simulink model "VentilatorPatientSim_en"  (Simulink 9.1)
settings: Solver=ode3  StartTime=0.0  StopTime=45  FixedStep=0.0001  RelTol=1e-3  EnableMultiTasking=on
undefined symbols (not defined in the file or in its folder): sgn

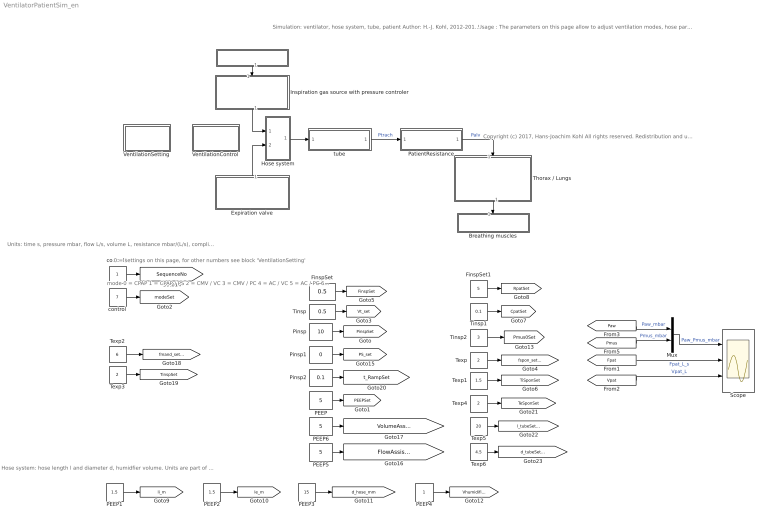
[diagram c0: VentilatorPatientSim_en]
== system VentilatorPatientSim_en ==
  note: Usage : The parameters on this page allow to adjust ventilation modes, hose parameters and patient properties. SequenceNo can select preprogrammed sequences. Suggestions : - place monitors at signals of interest - program a leak simulation and a leak compensation by the ventilator
  note: Copyright (c) 2017, Hans-Joachim Kohl All rights reserved. Redistribution and use in source and binary forms, with or without modification, are permitted provided that the following conditions are met: 1. Redistributions of source code must retain the above copyright notice, this list of conditions and the following disclaimer. 2. Redistributions in binary form must reproduce the above copyright notice, this list of conditions and the following disclaimer in the documentation and/or other materials provided with the distribution. THIS SOFTWARE IS PROVIDED BY THE COPYRIGHT HOLDERS AND CONTRIBUTORS "AS IS" AND ANY EXPRESS OR IMPLIED WARRANTIES, INCLUDING, BUT NOT LIMITED TO, THE IMPLIED WARRANTIES OF MERCHANTABILITY AND FITNESS FOR A PARTICULAR PURPOSE ARE DISCLAIMED. IN NO EVENT SHALL THE COPYRIGHT OWNER OR CONTRIBUTORS BE LIABLE FOR ANY DIRECT, INDIRECT, INCIDENTAL, SPECIAL, EXEMPLARY, OR CONSEQUENTIAL DAMAGES (INCLUDING, BUT NOT LIMITED TO, PROCUREMENT OF SUBSTITUTE GOODS OR SERVICES; LOSS OF USE, DATA, OR PROFITS; OR BUSINESS INTERRUPTION) HOWEVER CAUSED AND ON ANY THEORY OF LIABILITY, WHETHER IN CONTRACT, STRICT LIABILITY, OR TORT (INCLUDING NEGLIGENCE OR OTHERWISE) ARISING IN ANY WAY OUT OF THE USE OF THIS SOFTWARE, EVEN IF ADVISED OF THE POSSIBILITY OF SUCH DAMAGE. This is a simplified BSD license.
  note: Units: time s, pressure mbar, flow L/s, volume L, resistance mbar/(L/s), compliance L/mbar
  note: Hose system: hose length l and diameter d, humidfier volume. Units are part of the name.
  note: 0 = settings on this page, for other numbers see block 'VentilationSetting'
  note: mode 0 = CPAP 1 = CPAP / PS 2 = CMV / VC 3 = CMV / PC 4 = AC / VC 5 = AC / PC 6 = SIMV / VC 7 = SIMV / PC 8 = CPAP / ATC 9 = CPAP / PPS
  note: Simulation: ventilator, hose system, tube, patient Author: H.-J. Kohl, 2012-2019. Translation of a contribution 'Künstliche Beatmung' in 'Medizintechnische Systeme, ('Artificial Ventilation' in 'Medical Technology Systems') Springer Vieweg, ISBN 978-3-642-41238-7. The figures about ventilation modes have been created with this simulation. Technical details of the simulation are explained in a translated version of the contribution. Tested with Matlab 2017a
  " " : Subsystem
  Breathing muscles : Subsystem
  Expiration valve : Subsystem
  FinspSet : Constant  Value=0.5
  FinspSet1 : Constant  Value=5
  Hose system : Subsystem
  Inspiration gas source with pressure controler : Subsystem
  Mux : Mux  Inputs=2
  PEEP : Constant  Value=5
  PEEP1 : Constant  Value=1.5
  PEEP2 : Constant  Value=1.5
  PEEP3 : Constant  Value=15
  PEEP4 : Constant
  PEEP5 : Constant  Value=5
  PEEP6 : Constant  Value=5
  PatientResistance : Subsystem
  Pinsp : Constant  Value=10
  Pinsp1 : Constant  Value=0
  Pinsp2 : Constant  Value=0.1
  Scope : Scope  NumInputPorts=3
  Texp : Constant  Value=2
  Texp1 : Constant  Value=1.5
  Texp2 : Constant  Value=6
  Texp3 : Constant  Value=2
  Texp4 : Constant  Value=2
  Texp5 : Constant  Value=20
  Texp6 : Constant  Value=4.5
  Thorax / Lungs : Subsystem
  Tinsp : Constant  Value=0.5
  Tinsp1 : Constant  Value=0.1
  Tinsp2 : Constant  Value=3
  VentilationControl : Subsystem
  VentilationSetting : Subsystem
  control : Constant  Value=7  OutDataTypeStr=uint8
  control1 : Constant  OutDataTypeStr=uint32  SampleTime=0.0001
  tube : Subsystem
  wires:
  Thorax / Lungs/1(Pmus) -> Breathing muscles/1(" ")
  PatientResistance/1(" ") -> Thorax / Lungs/1(Palv)  "Palv"
  Pinsp/1 -> [PinspSet]
  PEEP/1 -> [PEEPSet]
  control/1 -> [modeSet]
  Tinsp/1 -> [Vt_set]
  Texp/1 -> [fspon_set_bpm]
  FinspSet/1 -> [FinspSet]
  Texp1/1 -> [TiSponSet]
  Tinsp1/1 -> [CpatSet]
  FinspSet1/1 -> [RpatSet]
  Inspiration gas source with pressure controler/1(Finsp) -> Hose system/1("   ")
  Expiration valve/1(" sValve") -> Hose system/2(" ")
  Hose system/1(Paw) -> tube/1(Paw)
  PEEP1/1 -> [li_m]
  PEEP2/1 -> [le_m]
  PEEP3/1 -> [d_hose_mm]
  PEEP4/1 -> [Vhumidifier_L]
  Tinsp2/1 -> [Pmus0Set]
  control1/1 -> [SequenceNo]
  Pinsp1/1 -> [PS_set]
  PEEP5/1 -> [FlowAssistSet_mbar__L_s]
  PEEP6/1 -> [VolumeAssistSet_mbar_L]
  Texp2/1 -> [fmand_set_bpm]
  Texp3/1 -> [TinspSet]
  Pinsp2/1 -> [t_RampSet]
  Texp4/1 -> [TeSponSet]
  tube/1(" ") -> PatientResistance/1(Ptrach)  "Ptrach"
  Texp5/1 -> [l_tubeSet_cm]
  Texp6/1 -> [d_tubeSet_mm]
  " "/1(" ") -> Inspiration gas source with pressure controler/1(" ")
  [Fpat] -> Scope/2  "Fpat_L_s"
  [Vpat] -> Scope/3  "Vpat_L"
  Mux/1 -> Scope/1  "Paw_Pmus_mbar"
  [Paw] -> Mux/1  "Paw_mbar"
  [Pmus] -> Mux/2  "Pmus_mbar"

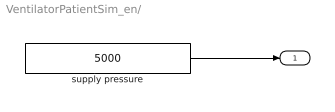
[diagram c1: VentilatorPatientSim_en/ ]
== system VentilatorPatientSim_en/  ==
  supply pressure : Constant  Value=5000
  " " : Outport
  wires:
  supply pressure/1 -> " "/1

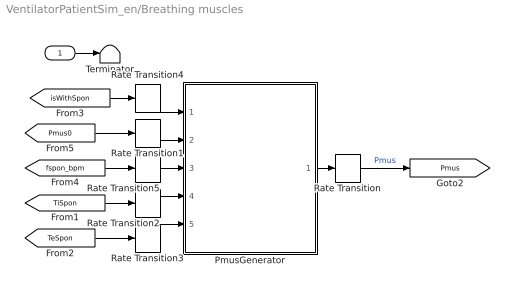
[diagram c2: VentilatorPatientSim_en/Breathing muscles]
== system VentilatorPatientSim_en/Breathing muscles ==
  " " : Inport
  PmusGenerator : Stateflow chart  TreatAsAtomicUnit=on
  Rate Transition{,1..5} (6 alike) : RateTransition  Integrity=off  Deterministic=off
  Terminator : Terminator
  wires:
  " "/1 -> Terminator/1
  PmusGenerator/1(Pmus) -> Rate Transition/1
  [TiSpon] -> Rate Transition2/1
  [TeSpon] -> Rate Transition3/1
  [Pmus0] -> Rate Transition1/1
  Rate Transition/1 -> [Pmus]  "Pmus"
  Rate Transition1/1 -> PmusGenerator/2(Pmus0)
  Rate Transition2/1 -> PmusGenerator/4(TiSpon)
  Rate Transition3/1 -> PmusGenerator/5(TeSpon)
  [isWithSpon] -> Rate Transition4/1
  Rate Transition4/1 -> PmusGenerator/1(isWithSpon)
  [fspon_bpm] -> Rate Transition5/1
  Rate Transition5/1 -> PmusGenerator/3(fspon_bpm)

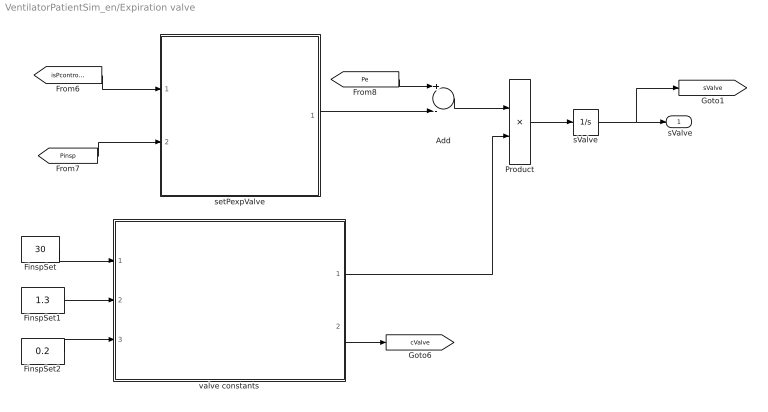
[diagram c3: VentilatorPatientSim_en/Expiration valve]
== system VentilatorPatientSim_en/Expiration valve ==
  Add : Sum  Inputs=+-
  FinspSet : Constant  Value=30
  FinspSet1 : Constant  Value=1.3
  FinspSet2 : Constant  Value=0.2
  Product : Product  Inputs=**
  sValve : Integrator  LimitOutput=on  UpperSaturationLimit=3  LowerSaturationLimit=0  ContinuousStateAttributes='sVentil'
  setPexpValve : Stateflow chart  TreatAsAtomicUnit=on
  valve constants : Stateflow chart  TreatAsAtomicUnit=on
  " sValve" : Outport
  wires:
  [isPcontrolled] -> setPexpValve/1(isPcontrolled)
  [Pinsp] -> setPexpValve/2(Pinsp)
  sValve/1 -> " sValve"/1, [sValve]
  [Pe] -> Add/1
  setPexpValve/1(PexpValve) -> Add/2
  Product/1 -> sValve/1
  Add/1 -> Product/1
  valve constants/1(cValve_sdot_mm_s__mbar) -> Product/2
  valve constants/2(cValve_flow_L_s__mm___mbar05) -> [cValve]
  FinspSet/1 -> valve constants/1(D_Valve_mm)
  FinspSet1/1 -> valve constants/2(rhoAir_kg_m3)
  FinspSet2/1 -> valve constants/3(tau3mm_s)

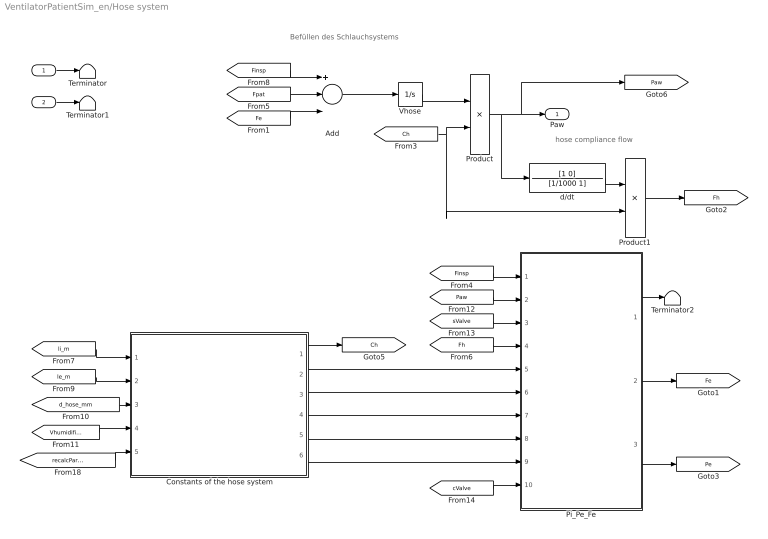
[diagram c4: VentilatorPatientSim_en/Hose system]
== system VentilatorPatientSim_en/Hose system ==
  note: Befüllen des Schlauchsystems
  note: hose compliance flow
  "   " : Inport
  " " : Inport  Port=2
  Add : Sum  Inputs=+--
  Constants of the hose system : Stateflow chart  TreatAsAtomicUnit=on
  Pi_Pe_Fe : Stateflow chart  TreatAsAtomicUnit=on
  Product : Product  Inputs=*/
  Product1 : Product
  Terminator : Terminator
  Terminator1 : Terminator
  Terminator2 : Terminator
  Vhose : Integrator
  d/dt : TransferFcn  Numerator=[1 0]  Denominator=[1/1000 1]
  Paw : Outport
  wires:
  "   "/1 -> Terminator/1
  " "/1 -> Terminator1/1
  [Finsp] -> Add/1
  Vhose/1 -> Product/1
  [Ch] -> Product/2, Product1/2
  Product/1 -> Paw/1, [Paw], d/dt/1
  Product1/1 -> [Fh]
  [Finsp] -> Pi_Pe_Fe/1(Finsp)
  [Fh] -> Pi_Pe_Fe/4(Fh)
  Pi_Pe_Fe/1(Pi) -> Terminator2/1
  Pi_Pe_Fe/2(Fe) -> [Fe]
  Pi_Pe_Fe/3(Pe) -> [Pe]
  Constants of the hose system/2(i_ie_Ch) -> Pi_Pe_Fe/5(i_ie_Ch)
  [li_m] -> Constants of the hose system/1(Li_m)
  [le_m] -> Constants of the hose system/2(Le_m)
  [d_hose_mm] -> Constants of the hose system/3(d_hose_mm)
  [Vhumidifier_L] -> Constants of the hose system/4(Vhumidifier_L)
  Constants of the hose system/1(Ch_L_mbar) -> [Ch]
  [Paw] -> Pi_Pe_Fe/2(Paw)
  Add/1 -> Vhose/1
  d/dt/1 -> Product1/1
  [sValve] -> Pi_Pe_Fe/3(sValve_mm)
  [cValve] -> Pi_Pe_Fe/10(cValve_L_s__mm___mbar05)
  Constants of the hose system/3(K1i_mbar__L_s) -> Pi_Pe_Fe/6(K1i)
  Constants of the hose system/4(K2i_mbar__L2_s2) -> Pi_Pe_Fe/7(K2i)
  Constants of the hose system/5(K1e_mbar__L_s) -> Pi_Pe_Fe/8(K1e)
  Constants of the hose system/6(K2e_mbar__L2_s2) -> Pi_Pe_Fe/9(K2e)
  [recalcParameters] -> Constants of the hose system/5(recalcParameters)
  [Fe] -> Add/3
  [Fpat] -> Add/2

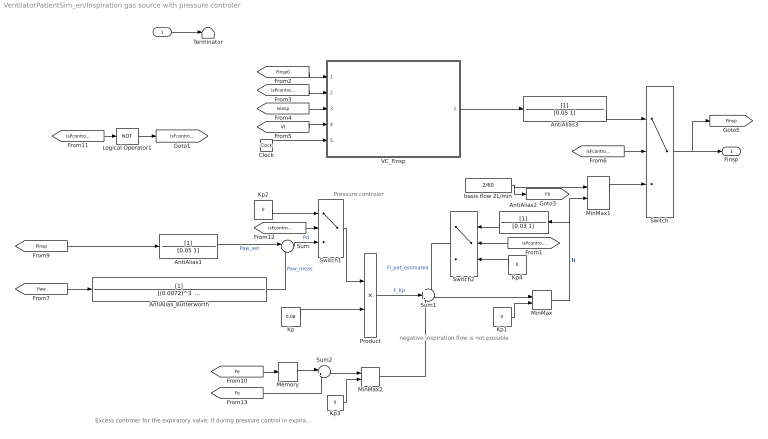
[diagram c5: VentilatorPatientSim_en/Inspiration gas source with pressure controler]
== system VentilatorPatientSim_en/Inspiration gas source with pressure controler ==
  note: Pressure controler
  note: Excess controler for the expiratory valve: If during pressure control in expirationthe the flow is greater than the basis flow, then Finsp is reduced to basis flow.
  note: negative inspiration flow is not possible
  " " : Inport
  AntiAlias1 : TransferFcn  Denominator=[0.05 1]
  AntiAlias2 : TransferFcn  Denominator=[0.03 1]
  AntiAlias3 : TransferFcn  Denominator=[0.05 1]
  AntiAlias_Butterworth : TransferFcn  Denominator="[(0.0072)^3   2*(0.0072)^2    2*0.0072   1]"
  Clock : Clock
  Kp : Constant  Value=0.08
  Kp{1..4} (4 alike) : Constant  Value=0
  Logical Operator1 : Logic  Operator=NOT  AllPortsSameDT=off  OutDataTypeStr=boolean
  Memory : Memory
  MinMax : MinMax  Function=max  Inputs=2
  MinMax1 : MinMax  Function=max  Inputs=2
  MinMax2 : MinMax  Function=max  Inputs=2
  Product : Product
  Sum : Sum  Inputs=|+-
  Sum1 : Sum  Inputs=++-
  Sum2 : Sum  Inputs=|+-
  Switch : Switch  Criteria=u2 ~= 0  ZeroCross=off
  Switch1 : Switch  Criteria=u2 ~= 0  ZeroCross=off
  Switch2 : Switch  Criteria=u2 ~= 0
  Terminator : Terminator
  VC_Finsp : Stateflow chart  TreatAsAtomicUnit=on
  basis flow 2L/min : Constant  Value=2/60
  Finsp : Outport
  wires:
  " "/1 -> Terminator/1
  [Finsp0] -> VC_Finsp/1(Finsp0)
  [isPcontrolled] -> VC_Finsp/2(isPcontrolled)
  [isInsp] -> VC_Finsp/3(isInsp)
  [Vt] -> VC_Finsp/4(Vt)
  Clock/1 -> VC_Finsp/5(time)
  VC_Finsp/1(Finsp) -> AntiAlias3/1
  Switch/1 -> Finsp/1, [Finsp]
  [Paw] -> AntiAlias_Butterworth/1
  [Pinsp] -> AntiAlias1/1
  Kp/1 -> Product/2
  Sum1/1 -> MinMax/1
  MinMax/1 -> MinMax1/2, AntiAlias2/1  "Fi"
  Kp1/1 -> MinMax/2
  Switch2/1 -> Sum1/1  "Fi_pat_estimated"
  Product/1 -> Sum1/2  "F_Kp"
  AntiAlias3/1 -> Switch/1
  MinMax1/1 -> Switch/3
  basis flow 2L/min/1 -> MinMax1/1, [Fb]
  [isPcontrolled] -> Logical Operator1/1
  Logical Operator1/1 -> [isFcontrolled]
  [isFcontrolled] -> Switch/2
  Kp2/1 -> Switch1/1
  [isFcontrolled] -> Switch1/2
  Sum/1 -> Switch1/3  "Pd"
  Switch1/1 -> Product/1
  AntiAlias1/1 -> Sum/1  "Paw_set"
  [Fe] -> Memory/1
  [Fb] -> Sum2/2
  Sum2/1 -> MinMax2/1
  Kp3/1 -> MinMax2/2
  MinMax2/1 -> Sum1/3
  Memory/1 -> Sum2/1
  AntiAlias2/1 -> Switch2/1
  [isPcontrolled] -> Switch2/2
  Kp4/1 -> Switch2/3
  AntiAlias_Butterworth/1 -> Sum/2  "Paw_meas"

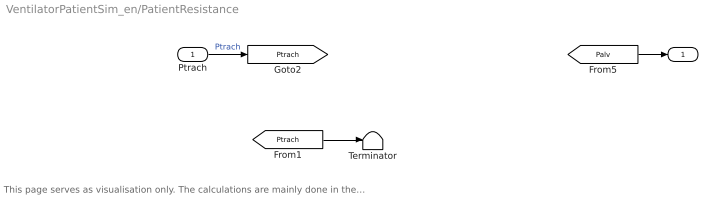
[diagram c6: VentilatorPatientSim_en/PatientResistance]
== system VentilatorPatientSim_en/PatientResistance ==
  note: This page serves as visualisation only. The calculations are mainly done in the block 'tube'
  Ptrach : Inport
  Terminator : Terminator
  " " : Outport
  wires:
  [Palv] -> " "/1
  Ptrach/1 -> [Ptrach]  "Ptrach"
  [Ptrach] -> Terminator/1

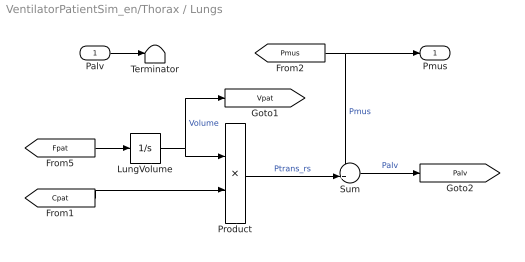
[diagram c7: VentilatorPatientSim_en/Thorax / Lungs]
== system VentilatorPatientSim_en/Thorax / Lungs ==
  Palv : Inport
  LungVolume : Integrator  ZeroCross=off  ContinuousStateAttributes='LungVolume'
  Product : Product  Inputs=*/
  Sum : Sum  Inputs=++|
  Terminator : Terminator
  Pmus : Outport
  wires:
  [Fpat] -> LungVolume/1
  LungVolume/1 -> Product/1, [Vpat]  "Volume"
  [Cpat] -> Product/2
  Palv/1 -> Terminator/1
  [Pmus] -> Pmus/1, Sum/1  "Pmus"
  Product/1 -> Sum/2  "Ptrans_rs"
  Sum/1 -> [Palv]  "Palv"

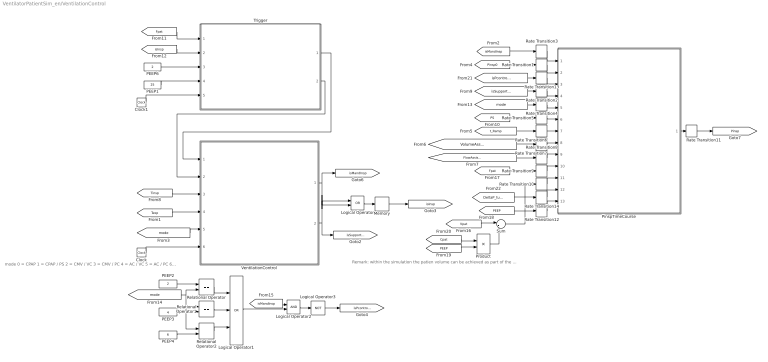
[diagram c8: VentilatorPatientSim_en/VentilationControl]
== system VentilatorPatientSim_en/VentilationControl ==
  note: Remark: within the simulation the patien volume can be achieved as part of the simulation data. Within a ventilator it is necessary to perform a volume integration with the measured patient flow.
  note: mode 0 = CPAP 1 = CPAP / PS 2 = CMV / VC 3 = CMV / PC 4 = AC / VC 5 = AC / PC 6 = SIMV / VC 7 = SIMV / PC 8 = CPAP / ATC 9 = CPAP / PPS
  Clock : Clock
  Clock1 : Clock
  Logical Operator : Logic  Operator=OR  AllPortsSameDT=off  OutDataTypeStr=boolean
  Logical Operator1 : Logic  Operator=OR  Inputs=3  AllPortsSameDT=off  OutDataTypeStr=boolean
  Logical Operator2 : Logic  AllPortsSameDT=off  OutDataTypeStr=boolean
  Logical Operator3 : Logic  Operator=NOT  AllPortsSameDT=off  OutDataTypeStr=boolean
  Memory : Memory
  PEEP1 : Constant  Value=25
  PEEP2 : Constant  Value=2
  PEEP3 : Constant  Value=4
  PEEP4 : Constant  Value=6
  PEEP6 : Constant  Value=2
  PinspTimeCourse : Stateflow chart  TreatAsAtomicUnit=on
  Product : Product
  Rate Transition{1..14} (14 alike) : RateTransition  Integrity=off  Deterministic=off
  Relational Operator : RelationalOperator  Operator===  OutDataTypeStr=boolean
  Relational Operator1 : RelationalOperator  Operator===  OutDataTypeStr=boolean
  Relational Operator2 : RelationalOperator  Operator===  OutDataTypeStr=boolean
  Sum : Sum  Inputs=|+-
  Trigger : Stateflow chart  TreatAsAtomicUnit=on
  VentilationControl : Stateflow chart  TreatAsAtomicUnit=on
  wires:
  Trigger/1(isInspTrigger) -> VentilationControl/1(isInspTrigger)
  Trigger/2(isExpTrigger) -> VentilationControl/2(isExpTrigger)
  [mode] -> VentilationControl/5(mode)
  [t_Ramp] -> Rate Transition6/1
  [VolumeAssist_mbar_L] -> Rate Transition7/1
  [FlowAssist_mbar__L_s] -> Rate Transition8/1
  [PS] -> Rate Transition5/1
  VentilationControl/1(isMandInsp) -> [isMandInsp], Logical Operator/1
  [Fpat] -> Trigger/1(Fpat)
  PinspTimeCourse/1(Pinsp) -> Rate Transition11/1
  [Tinsp] -> VentilationControl/3(Tinsp)
  [Texp] -> VentilationControl/4(Texp)
  [isMandInsp] -> Rate Transition3/1
  VentilationControl/2(isSupportedInsp) -> [isSupportedInsp], Logical Operator/2
  [Pinsp0] -> Rate Transition1/1
  [isSupportedInsp] -> Rate Transition2/1
  [mode] -> Rate Transition4/1
  PEEP6/1 -> Trigger/3(FinspTrigger_lpm)
  PEEP1/1 -> Trigger/4(FpercentExpTrigger)
  [isInsp] -> Trigger/2(isInsp)
  Logical Operator/1 -> Memory/1
  [mode] -> Relational Operator/2, Relational Operator1/1, Relational Operator2/1
  Relational Operator/1 -> Logical Operator1/1
  Relational Operator1/1 -> Logical Operator1/2
  [isMandInsp] -> Logical Operator2/1
  Logical Operator1/1 -> Logical Operator2/2
  Logical Operator2/1 -> Logical Operator3/1
  Logical Operator3/1 -> [isPcontrolled]
  PEEP2/1 -> Relational Operator/1
  PEEP3/1 -> Relational Operator1/2
  Clock/1 -> VentilationControl/6(time)
  [Fpat] -> Rate Transition9/1
  Rate Transition3/1 -> PinspTimeCourse/1(isMandInsp)
  Rate Transition1/1 -> PinspTimeCourse/2(PinspSet)
  Rate Transition2/1 -> PinspTimeCourse/4(isSuppInsp)
  Rate Transition4/1 -> PinspTimeCourse/5(mode)
  Rate Transition5/1 -> PinspTimeCourse/6(PS)
  Rate Transition6/1 -> PinspTimeCourse/7(t_Rampe)
  Rate Transition7/1 -> PinspTimeCourse/8(dP_dV)
  Rate Transition8/1 -> PinspTimeCourse/9(dP_dFlow)
  Rate Transition9/1 -> PinspTimeCourse/10(Fpat)
  Rate Transition10/1 -> PinspTimeCourse/11(Vpat)
  Rate Transition11/1 -> [Pinsp]
  [PEEP] -> Rate Transition12/1
  Rate Transition12/1 -> PinspTimeCourse/13(Peep)
  Memory/1 -> [isInsp]
  Clock1/1 -> Trigger/5(time)
  [Vpat] -> Sum/1
  Product/1 -> Sum/2
  [PEEP] -> Product/2
  [Cpat] -> Product/1
  Sum/1 -> Rate Transition10/1
  Rate Transition13/1 -> PinspTimeCourse/3(isPcontrolled)
  [isPcontrolled] -> Rate Transition13/1
  PEEP4/1 -> Relational Operator2/2
  Relational Operator2/1 -> Logical Operator1/3
  Rate Transition14/1 -> PinspTimeCourse/12(DeltaP_tube)
  [DeltaP_tube] -> Rate Transition14/1

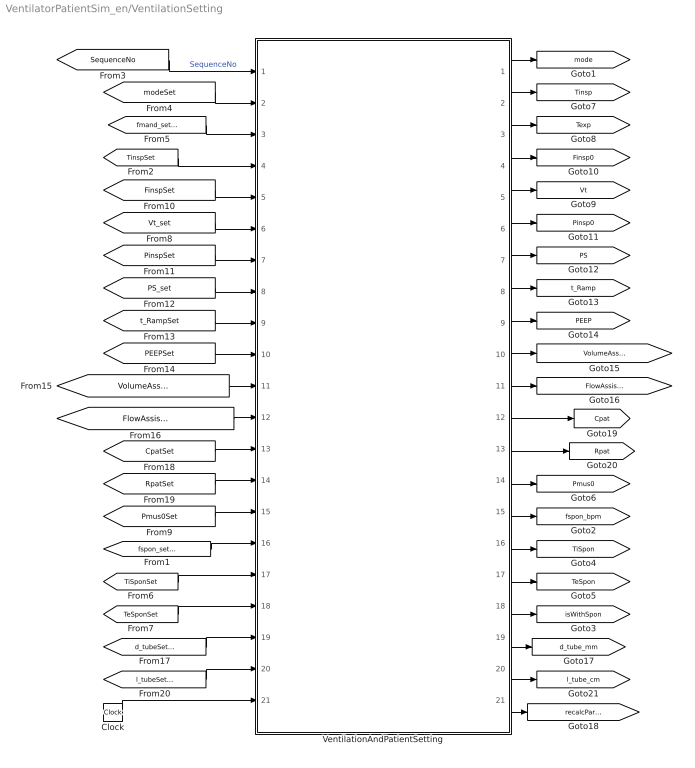
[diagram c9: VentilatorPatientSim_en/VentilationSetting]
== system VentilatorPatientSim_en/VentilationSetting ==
  Clock : Clock
  VentilationAndPatientSetting : Stateflow chart  TreatAsAtomicUnit=on
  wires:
  [SequenceNo] -> VentilationAndPatientSetting/1(SequenceNo)  "SequenceNo"
  VentilationAndPatientSetting/1(mode) -> [mode]
  [modeSet] -> VentilationAndPatientSetting/2(modeSet)
  [fmand_set_bpm] -> VentilationAndPatientSetting/3(f_set_bpm)
  [TinspSet] -> VentilationAndPatientSetting/4(TinspSet)
  VentilationAndPatientSetting/18(isWithSpon) -> [isWithSpon]
  VentilationAndPatientSetting/16(TiSpon) -> [TiSpon]
  VentilationAndPatientSetting/17(TeSpon) -> [TeSpon]
  VentilationAndPatientSetting/14(Pmus0) -> [Pmus0]
  VentilationAndPatientSetting/2(Tinsp) -> [Tinsp]
  VentilationAndPatientSetting/3(Texp) -> [Texp]
  [fspon_set_bpm] -> VentilationAndPatientSetting/16(fspon_set_bpm)
  [TiSponSet] -> VentilationAndPatientSetting/17(TiSponSet)
  [Pmus0Set] -> VentilationAndPatientSetting/15(Pmus0Set)
  Clock/1 -> VentilationAndPatientSetting/21(time)
  [TeSponSet] -> VentilationAndPatientSetting/18(TeSponSet)
  VentilationAndPatientSetting/15(fspon_bpm) -> [fspon_bpm]
  [Vt_set] -> VentilationAndPatientSetting/6(Vt_set)
  [FinspSet] -> VentilationAndPatientSetting/5(FinspSet)
  VentilationAndPatientSetting/5(Vt) -> [Vt]
  VentilationAndPatientSetting/4(Finsp0) -> [Finsp0]
  [PinspSet] -> VentilationAndPatientSetting/7(PinspSet)
  [PS_set] -> VentilationAndPatientSetting/8(PS_set)
  [t_RampSet] -> VentilationAndPatientSetting/9(t_RampSet)
  [PEEPSet] -> VentilationAndPatientSetting/10(PEEPSet)
  [VolumeAssistSet_mbar_L] -> VentilationAndPatientSetting/11(VolumeAssistSet_mbar_L)
  [FlowAssistSet_mbar__L_s] -> VentilationAndPatientSetting/12(FlowAssistSet_mbar__L_s)
  VentilationAndPatientSetting/6(Pinsp0) -> [Pinsp0]
  VentilationAndPatientSetting/7(PS) -> [PS]
  VentilationAndPatientSetting/8(t_Ramp) -> [t_Ramp]
  VentilationAndPatientSetting/9(PEEP) -> [PEEP]
  VentilationAndPatientSetting/10(VolumeAssist_mbar_L) -> [VolumeAssist_mbar_L]
  VentilationAndPatientSetting/11(FlowAssist_mbar__L_s) -> [FlowAssist_mbar__L_s]
  [d_tubeSet_mm] -> VentilationAndPatientSetting/19(d_tubeSet_mm)
  VentilationAndPatientSetting/19(d_tube_mm) -> [d_tube_mm]
  VentilationAndPatientSetting/21(recalcParameters) -> [recalcParameters]
  [CpatSet] -> VentilationAndPatientSetting/13(CpatSet)
  [RpatSet] -> VentilationAndPatientSetting/14(RpatSet)
  [l_tubeSet_cm] -> VentilationAndPatientSetting/20(l_tubeSet_cm)
  VentilationAndPatientSetting/20(l_tube_cm) -> [l_tube_cm]
  VentilationAndPatientSetting/12(Cpat) -> [Cpat]
  VentilationAndPatientSetting/13(Rpat) -> [Rpat]

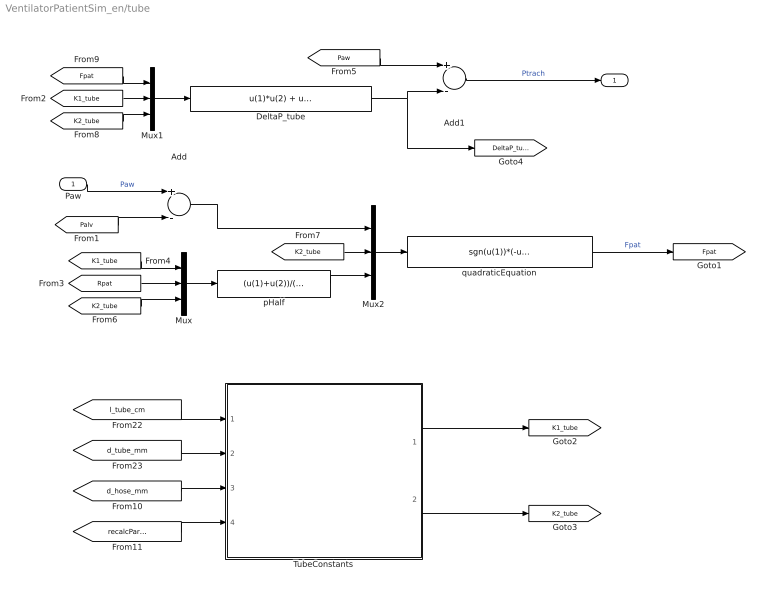
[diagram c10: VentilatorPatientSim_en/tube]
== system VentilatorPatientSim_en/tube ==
  Paw : Inport
  Add : Sum  Inputs=+-
  Add1 : Sum  Inputs=+-
  DeltaP_tube : Fcn  Expr=u(1)*u(2) + u(1)*abs(u(1))*u(3)
  Mux : Mux  Inputs=3
  Mux1 : Mux  Inputs=3
  Mux2 : Mux  Inputs=3
  TubeConstants : Stateflow chart  TreatAsAtomicUnit=on
  pHalf : Fcn  Expr=(u(1)+u(2))/(2*u(3))
  quadraticEquation : Fcn  Expr=sgn(u(1))*(-u(3)+sqrt(u(3)^2+abs(u(1))/u(2)))
  " " : Outport
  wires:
  quadraticEquation/1 -> [Fpat]  "Fpat"
  [Palv] -> Add/2
  Paw/1 -> Add/1  "Paw"
  Add/1 -> Mux2/1
  Mux/1 -> pHalf/1
  [K1_tube] -> Mux/1
  [Rpat] -> Mux/2
  [K2_tube] -> Mux/3
  pHalf/1 -> Mux2/3
  [K2_tube] -> Mux2/2
  Mux2/1 -> quadraticEquation/1
  Mux1/1 -> DeltaP_tube/1
  [Fpat] -> Mux1/1
  [K1_tube] -> Mux1/2
  [K2_tube] -> Mux1/3
  Add1/1 -> " "/1  "Ptrach"
  [Paw] -> Add1/1
  DeltaP_tube/1 -> Add1/2, [DeltaP_tube]
  [l_tube_cm] -> TubeConstants/1(l_tube_cm)
  [d_tube_mm] -> TubeConstants/2(d_tube_mm)
  TubeConstants/1(K1_tube_mbar__L_s) -> [K1_tube]
  TubeConstants/2(K2_tube_mbar__L2_s2) -> [K2_tube]
  [d_hose_mm] -> TubeConstants/3(d_hose_mm)
  [recalcParameters] -> TubeConstants/4(recalcParameters)

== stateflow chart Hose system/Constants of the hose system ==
  state CalculateHoseParameters/
    entry:
    mm_ = 1./1000; cm_ = 1./100; L_ = 1./1000;  mbar_ = 100.; min_ = 60.; s_=1.;
    A = (3.1416/4)*(d_hose_mm*mm_)^2;
    V_i = A * Li_m + Vhumidifier_L * L_;
    V_e = A * Le_m ;
    Ch = (V_i + V_e) / (1013*mbar_);
    i_ie_Ch = V_i / (V_i + V_e);
    K1i = 0.696*mbar_/(L_/s_)*(10/d_hose_mm)^4*Li_m;
    Ffix =Li_m^-0.571*(d_hose_mm/10)^2.741*250*L_/min_;
    K2i =  (38.8*mbar_/Ffix - K1i) / Ffix;
    K1e =0.696*mbar_/(L_/s_)*(10/d_hose_mm)^4*Le_m;
    Ffix =Le_m^-0.571*(d_hose_mm/10)^2.741*250*L_/min_;
    K2e = (38.8*mbar_/Ffix - K1e) / Ffix;
    Ch_L_mbar            = Ch / (L_/mbar_);
    K1e_mbar__L_s     = K1e / (mbar_/(L_/s_));
    K2e_mbar__L2_s2 = K2e / (mbar_/(L_/s_)^2);
    K1i_mbar__L_s      = K1i / (mbar_/(L_/s_));
    K2i_mbar__L2_s2  = K2i / (mbar_/(L_/s_)^2);
  (default) -> CalculateHoseParameters
  CalculateHoseParameters -> CalculateHoseParameters : [recalcParameters]

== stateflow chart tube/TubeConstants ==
  state Tube/
    % Calculations are done in SI-base units
    entry:
    mm_ = 1./1000; cm_ = 1./100; L_ = 1./1000; mbar_ = 100.; min_ = 60.; s_=1.;
    d_tube_by_d_trach = 0.6;
    A_tube = (3.1416/4)*(d_tube_mm*mm_)^2;
    A_hose = (3.1416/4)*(d_hose_mm*mm_)^2;
    A_trachea = (3.1416/4)*(d_tube_mm*mm_/d_tube_by_d_trach)^2;
    rho = 1.21;% kg/m^3
    A2_by_A1 = A_tube / A_hose;
    Psi = 0.615+0.018*A2_by_A1+0.1007*A2_by_A1^2+0.2662*A2_by_A1^3;
    zeta2 = 1.5*((1-Psi)/Psi)^2;
    K2_s_t = zeta2*(rho/2) / A_tube^2;
    zeta1 = (1 - A_tube / A_trachea)^2;
    K2_t_t =  zeta1*(rho/2) / A_trachea^2;
    K1_cyl= 0.696*mbar_/(L_/s_)*(10/d_tube_mm)^4*(l_tube_cm*cm_);
    Ffix = (l_tube_cm*cm_)^-0.571*(d_tube_mm/10)^2.741*250*L_/min_;
    K2_cyl = (38.8*mbar_/Ffix - K1_cyl) / Ffix;
    K1_tube_mbar__L_s = K1_cyl / (mbar_/(L_/s_));
    K2_tube_mbar__L2_s2 = (K2_cyl + K2_s_t + K2_t_t) / (mbar_/(L_/s_)^2);
  Tube -> Tube : [recalcParameters]

== stateflow chart Inspiration gas source
with
pressure controler/VC_Finsp ==
  state waitForInsp/
  state inspFlowTime/
    entry:
    Finsp = Finsp0;
    tnext = time + TinspFlow;
  state noFlow/
    entry:
    Finsp = 0;
  (default) -> noFlow : {TinspFlow = Vt / Finsp0;}
  waitForInsp -> inspFlowTime : [isInsp]
  noFlow -> waitForInsp : [ ! isInsp && ! isPcontrolled ]
  inspFlowTime -> noFlow : [time >= tnext || isPcontrolled]

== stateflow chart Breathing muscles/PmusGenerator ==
  state Apnoe/
  state Breathing/
    state insp/
      entry: t=0;
      entry,during:
      Pmus = -Pmus0 * (1-pow(2.7183,-5*t/TiSpon)) / (1-pow(2.7183,-5));
      t = t + 0.001;
    state exp/
      entry: t=0;
      entry,during:
      Pmus = -Pmus0 * (pow(2.7183,-4*t/TeSpon) - pow(2.7183,-4)) / (1-pow(2.7183,-4));
      t = t + 0.001;
    state expPause/
      entry:
      t=0;
      tpause =  60./fspon_bpm - TiSpon - TeSpon;
      entry,during:
      t = t + 0.001;
    (default) -> insp
    insp -> exp : [t > TiSpon]
    expPause -> insp : [t > tpause]
    exp -> expPause : [t > TeSpon]
  (default) -> Apnoe
  Breathing -> Apnoe : [! isWithSpon]
  Apnoe -> Breathing : [isWithSpon]

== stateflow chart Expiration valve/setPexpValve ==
  state Pcontrolled/
    entry,during:
    PexpValve = Pinsp;
  state Vcontrolled/
    entry:
    PexpValve = 100;
  Pcontrolled -> Vcontrolled : [ ! isPcontrolled]
  (default) -> Pcontrolled
  Vcontrolled -> Pcontrolled : [isPcontrolled]

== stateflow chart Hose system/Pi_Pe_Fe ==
  state calc_Pi_Pe_Fe/
    entry, during:
    Fhi = i_ie_Ch * Fh;
    Fhe = (Fh - Fhi);
    Pi = Paw + K1i * (Finsp - Fhi/2) + K2i * abs(Finsp - Fhi/2)*(Finsp - Fhi/2);
    fpp = sValve_mm * cValve_L_s__mm___mbar05;
    a = 1 + fpp^2 * K2e;
    b = (K1e - K2e * Fhe)*fpp;
    c = -Paw + K1e*Fhe/2 + K2e*(Fhe/2)^2;
    pHalf = b/(2*a);
    sqrt_Pe = -pHalf + (pHalf^2 - c/a)^0.5;
    Pe = sqrt_Pe^2;
    Fe = sqrt_Pe * sValve_mm * cValve_L_s__mm___mbar05;
  (default) -> calc_Pi_Pe_Fe

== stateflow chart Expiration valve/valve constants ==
  state calcValve/
    entry:
    cValve_sdot_mm_s__mbar            = (3 / tau3mm_s)/10;                                                           % at a pressure difference of 10mbar a movement over 3mm requires tau3mm_s
    cValve_flow_L_s__mm___mbar05 = D_Valve_mm * 3.1416 * sqrt( rhoAir_kg_m3 / 2) / 100;   % 1/100 = (mm/m) / ((L/cbm)/(mm/m)/(mbar/Pa)^0.5)
  (default) -> calcValve

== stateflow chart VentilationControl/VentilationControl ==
  state CPAP/
    entry:
    isMandInsp = 0;
    isSupportedInsp = 0;
    state PS/
      entry:
      isSupportedInsp = 1;
      exit:
      isSupportedInsp = 0;
    state noPS/
    (default) -> noPS
    noPS -> PS : [isInspTrigger && mode == 1]
    PS -> noPS : [isExpTrigger]
  state CMV/
    entry:
    isSupportedInsp = 0;
    state exp/
      entry:
      isMandInsp = 0;
      tnext = time + Texp;
    state insp/
      entry:
      isMandInsp = 1;
      tnext = time + Tinsp;
    (default) -> insp
    insp -> exp : [time >= tnext]
    exp -> insp : [time >= tnext]
  state AC_or_SIMV/
    entry:
    isSupportedInsp = 0;
    SyncDuration =  min( Texp-0.5, 5.0);
    tnextSync = time;
    tnextForce = tnextSync + SyncDuration;
    state waitForTriggerOrForced/
      entry:
      isAC = (mode == 4 || mode == 5);
    state MandStroke/
      entry:
      isMandInsp = 1;
      tnext = time + Tinsp;
      tnextSync = tnextSync + Tinsp + Texp;
      tnextForce = tnextSync + SyncDuration;
    state awaitProtectionTime/
      entry:
      isMandInsp = 0;
      tnext = time + 0.5;
    state allowSupport/
    state PS/
      entry:
      isSupportedInsp = 1;
      exit:
      isSupportedInsp = 0;
    (default) -> waitForTriggerOrForced
    (junction 165) -> waitForTriggerOrForced
    (junction 166) -> (junction 165)
    (junction 167) -> (junction 165) : [isAC]
    allowSupport -> (junction 166) : [time >= tnextSync]
    waitForTriggerOrForced -> MandStroke : [isInspTrigger || time >= tnextForce]
    MandStroke -> awaitProtectionTime : [time >= tnext]
    awaitProtectionTime -> (junction 167) : [time >= tnext]
    (junction 167) -> allowSupport
    PS -> awaitProtectionTime : [isExpTrigger]
    allowSupport -> PS : [isInspTrigger && time < tnextSync]
  (default) -> CPAP
  (junction 192) -> CPAP : [mode == 0 || mode == 1 || mode == 6]
  CPAP -> (junction 192) : [ ! (mode == 0 || mode == 1 || mode == 6)]
  (junction 192) -> CMV : [mode == 2 || mode == 3]
  CMV -> (junction 192) : [ ! (mode == 2 || mode == 3)]
  (junction 192) -> AC_or_SIMV : [ mode >= 4 && mode <= 7]
  AC_or_SIMV -> (junction 192) : [ ! (mode >= 4 && mode <= 7)]

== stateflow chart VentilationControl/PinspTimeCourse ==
  state MandInsp/
    entry:
    Pinsp = PinspSet;
    exit:
    Pinsp = Peep;
  state PS/
    entry:
    dP = PS * 0.001 / max( t_Rampe, 0.001);
    Pinsp = Peep + dP;
    during:
    Pinsp = min(Pinsp + dP, Peep + PS);
    exit:
    Pinsp = Peep;
  state CPAP_ATC/
    entry, during:
    Pinsp = Peep + DeltaP_tube;
    exit:
    Pinsp = Peep;
  state PPS/
    state PPS_exsp/
      entry: Pinsp = Peep;
      exit: V0 = Vpat;
    state PPS_insp/
      entry, during:
      Pinsp = Peep + max(Vpat - V0,0) * dP_dV + Fpat * dP_dFlow ;
      exit:
      Pinsp = Peep;
    PPS_insp -> PPS_exsp : [Fpat <= 0]
    PPS_exsp -> PPS_insp : [Fpat > 0]
    (default) -> PPS_exsp
  state exsp/
    entry: Pinsp = Peep;
  (junction 228) -> MandInsp : [isMandInsp && isPcontrolled]
  MandInsp -> (junction 228) : [ ! (isMandInsp && isPcontrolled)]
  (junction 228) -> PS : [isSuppInsp]
  (default) -> (junction 228)
  PS -> (junction 228) : [ ! isSuppInsp]
  (junction 228) -> exsp
  (junction 228) -> CPAP_ATC : [mode == 8]
  exsp -> (junction 228) : [(isMandInsp && isPcontrolled) || isSuppInsp || mode == 8 || mode == 9]
  CPAP_ATC -> (junction 228) : [ ! (mode == 8)]
  PPS -> (junction 228) : [ ! (mode == 9)]
  (junction 228) -> PPS : [mode == 9]

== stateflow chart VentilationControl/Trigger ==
  state insp/
    entry:
    FiMax = Fpat;
    during:
    FiMax = max(Fpat, FiMax);
  state exp_insp_is_triggered/
    entry:
    isInspTrigger = 1;
    tnext = time + 0.01;
  state switchToInsp/
    exit:
    isInspTrigger = 0;
  state exp/
  state insp_exp_is_triggered/
    entry:
    isExpTrigger = 1;
    tnext = time + 0.01;
  state switchToExp/
    exit:
    isExpTrigger = 0;
  state WaitForExpFlow/
  switchToInsp -> insp : [isInsp]
  exp_insp_is_triggered -> switchToInsp : [time >= tnext]
  switchToInsp -> (junction 260)
  exp -> exp_insp_is_triggered : [Fpat > FinspTrigger_lpm/60. && ! isInsp]
  (junction 258) -> insp
  exp -> (junction 258) : [isInsp]
  insp -> insp_exp_is_triggered : [Fpat < FiMax * FpercentExpTrigger/100. && isInsp]
  insp -> (junction 259) : [ ! isInsp]
  (junction 259) -> (junction 260)
  (junction 260) -> exp
  (default) -> exp : {FiMax=0;  isInspTrigger = 0;  isExpTrigger = 0;}
  switchToExp -> WaitForExpFlow : [! isInsp]
  insp_exp_is_triggered -> switchToExp : [time >= tnext]
  WaitForExpFlow -> exp : [Fpat < 0]

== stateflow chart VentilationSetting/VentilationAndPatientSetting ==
  state SchlauchFuellen/
    entry:
    tnext = time + 1.5;
    mode = 0;
    isWithSpon = 0;
    Tinsp = TinspSet;
    Texp = 60.0/f_set_bpm - Tinsp;
    fspon_bpm = fspon_set_bpm;
    TiSpon = TiSponSet;
    TeSpon = TeSponSet;
    Pmus0 = Pmus0Set;
    Finsp0 = FinspSet;
    Vt = Vt_set;
    PS = PS_set;
    Pinsp0 = PinspSet;
    t_Ramp = t_RampSet;
    PEEP = PEEPSet;
    VolumeAssist_mbar_L = VolumeAssistSet_mbar_L;
    FlowAssist_mbar__L_s = FlowAssistSet_mbar__L_s;
    Cpat = CpatSet;
    Rpat = RpatSet;
    d_tube_mm = d_tubeSet_mm;
    l_tube_cm = l_tubeSet_cm;
    recalcParameters = 0;
  state SetByParameters/
    entry:
    mode = modeSet;
    isWithSpon = 1;
  state CPAP/
    entry:
    tnext = time + 12;
    mode = 0;
    isWithSpon = 1;
    PEEP = 5;
    Cpat = 0.1;
    Rpat = 5;
    TiSpon = 1.3;
    TeSpon = 2.;
    fspon_bpm = 15;
    Pmus0 = 3;
    d_tube_mm = 4.5;
    l_tube_cm = 20;
    recalcParameters = 1;
  state CMV_VC/
    entry:
    tnext = time + 19;
    mode = 2;
    isWithSpon = 0;
    Tinsp = 2;
    f_bpm = 12;
    Texp = 60.0/f_bpm - Tinsp;
    Finsp0 = 0.5;
    Vt = 0.5;
    PEEP = 5;
    Cpat = 0.1;
    Rpat = 5;
    d_tube_mm = 8;
    l_tube_cm = 20;
    recalcParameters = 1;
  state VC_versus_PC/
    entry:
    tnext = time + 19;
    mode = 2;
    isWithSpon = 0;
    Tinsp = 2;
    f_bpm = 12;
    Texp = 60.0/f_bpm - Tinsp;
    Finsp0 = 0.5;
    Vt = 0.5;
    PEEP = 5;
    Cpat = 0.1;
    Rpat = 5;
    d_tube_mm = 30; % kein Tube
    l_tube_cm = 0;
    recalcParameters = 1;
  state simuliere3/
    entry:
    recalcParameters = 0;
  state simuliere1/
    entry:
    recalcParameters = 0;
  state simuliere4/
    entry:
    recalcParameters = 0;
  state AC_PC/
    entry:
    mode = 5;
    isWithSpon = 1;
    Pinsp0 = 10;
    TiSpon = 0.4;
    TeSpon = 0.4;
    fspon_bpm = 15;
    Pmus0 = 1.5;
  state CPAP_PS/
    entry:
    tnext = time + 8;
    mode = 1;
    PS = 5;
  state PC/
    entry:
    mode = 3;
    Pinsp0 = 10;
  state SIMV_PC/
    entry:
    mode = 7;
    isWithSpon = 1;
    Tinsp = 2;
    f_bpm = 6;
    Texp = 60.0/f_bpm - Tinsp;
    Pinsp0 = 10;
    PEEP = 5;
    PS = 0;
    Cpat = 0.1;
    Rpat = 5;
    TiSpon = 1.5;
    TeSpon = 2.0;
    fspon_bpm = 15;
    Pmus0 = 3;
    d_tube_mm = 8;
    l_tube_cm = 20;
    recalcParameters = 1;
  state CPAP_ATC/
    entry:
    tnext = time + 12;
    mode = 8;
  state simuliere2/
    entry:
    recalcParameters = 0;
  state CPAP_PPS/
    entry:
    tnext = time + 12;
    mode = 9;
  (default) -> SchlauchFuellen
  SchlauchFuellen -> (junction 336) : [time >= tnext]
  (junction 336) -> SetByParameters
  (junction 336) -> (junction 339) : [SequenceNo > 0]
  (junction 337) -> (junction 338)
  (junction 339) -> (junction 337) : [SequenceNo == 4]
  (junction 338) -> VC_versus_PC
  (junction 339) -> CMV_VC : [SequenceNo == 1]
  (junction 339) -> CPAP : [SequenceNo == 3]
  (junction 339) -> (junction 340)
  CPAP -> simuliere3
  VC_versus_PC -> simuliere4
  CMV_VC -> simuliere1
  simuliere3 -> CPAP_PS : [time > tnext]
  simuliere1 -> AC_PC : [time > tnext]
  simuliere4 -> PC : [time > tnext]
  CPAP_PS -> CPAP_ATC : [time > tnext]
  (junction 340) -> SIMV_PC : [ SequenceNo == 2]
  CPAP_ATC -> CPAP_PPS : [time > tnext]
  SIMV_PC -> simuliere2
